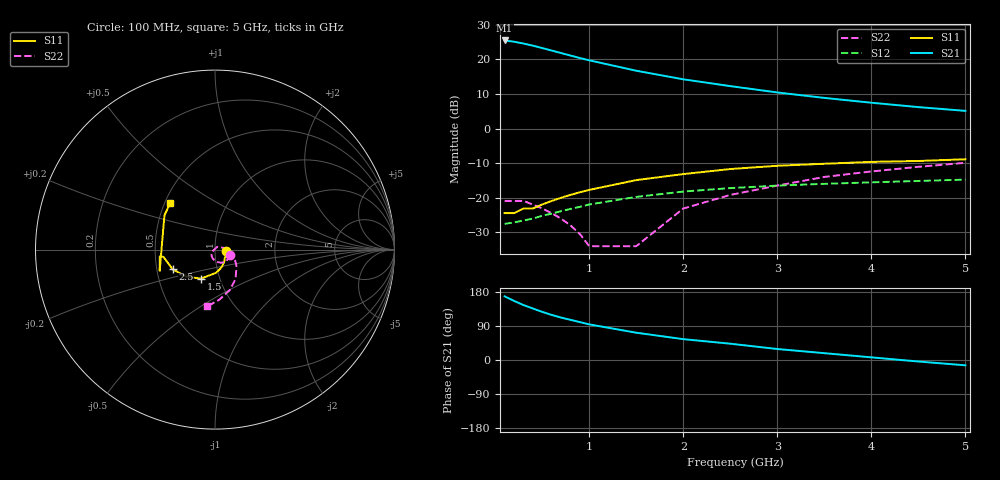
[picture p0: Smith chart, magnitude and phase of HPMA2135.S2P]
! HPMA-2135
! Typical S-Parameters, Z  = 50, T  = 25 C, I  = 25mA
# ghz s ma r 50
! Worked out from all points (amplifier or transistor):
!   18 points, 100 MHz to 5 GHz, reference 50 ohm
!   highest |S21| = 25.4 dB at 100 MHz (marker M1)
!   |S21| within 3 dB of that: start of sweep to 611.7 MHz
!   unconditionally stable (mu >= 1): start of sweep to end of sweep
!   at 400 MHz: K = 1.02, MAG = 24.1 dB, |S12| = -26.0 dB
!   at 1 GHz: K = 1.02, MAG = 20.0 dB, |S12| = -21.9 dB
!   at 5 GHz: K = 1.26, MAG = 6.9 dB, |S12| = -14.8 dB
!   S11 on the Smith chart (normalised r, x): 100 MHz: 1.13, -0.02; 1.5 GHz: 0.81, -0.27; 2.5 GHz: 0.61, -0.14; 5 GHz: 0.53, +0.32
0.1  0.06 -10.0  18.72 168.0  0.042 8.0  0.09 -18.0
0.2  0.06 -18.0  17.94 156.0  0.044 15.0  0.09 -34.0
0.3  0.07 -29.0  16.91 145.0  0.047 21.0  0.09 -50.0
0.4  0.07 -39.0  15.75 136.0  0.05 26.0  0.08 -66.0
0.5  0.08 -48.0  14.55 127.0  0.055 30.0  0.07 -80.0
0.6  0.09 -58.0  13.38 119.0  0.059 33.0  0.06 -93.0
0.7  0.1 -66.0  12.33 112.0  0.064 35.0  0.05 -106.0
0.8  0.11 -74.0  11.34 106.0  0.069 36.0  0.04 -118.0
0.9  0.12 -82.0  10.44 100.0  0.074 37.0  0.03 -133.0
1  0.13 -88.0  9.67 94.0  0.08 38.0  0.02 -146.0
1.5  0.18 -116.0  6.84 72.0  0.103 37.0  0.02 50.0
2  0.22 -137.0  5.14 55.0  0.123 33.0  0.07 5.0
2.5  0.26 -155.0  4.1 43.0  0.138 30.0  0.11 -17.0
3  0.29 -172.0  3.32 29.0  0.15 26.0  0.15 -37.0
3.5  0.31 -173.0  2.77 18.0  0.159 23.0  0.2 -55.0
4  0.33 -159.0  2.36 7.0  0.167 20.0  0.24 -70.0
4.5  0.34 146.0  2.04 -4.0  0.175 17.0  0.28 -85.0
5  0.36 134.0  1.8 -14.0  0.183 14.0  0.32 -98.0
